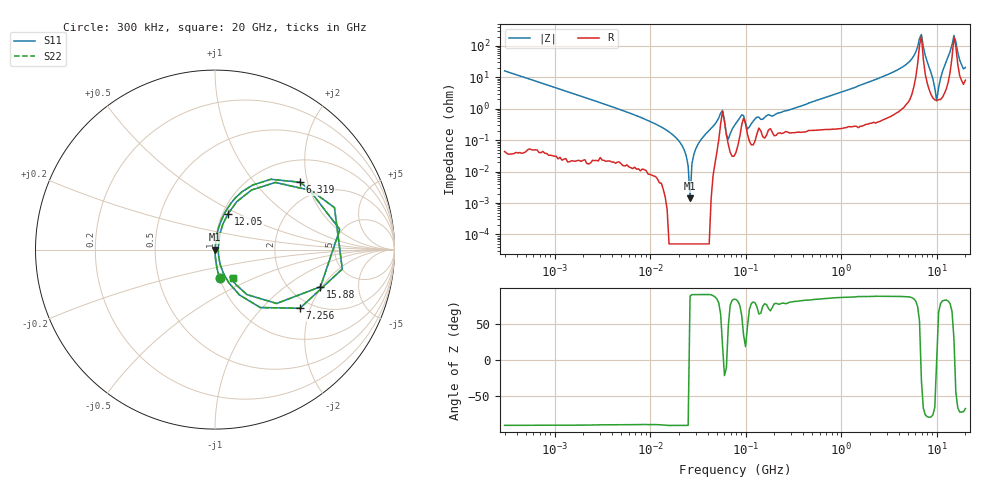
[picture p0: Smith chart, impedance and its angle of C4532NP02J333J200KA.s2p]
! S-parameter Generated by TDK Corporation
! Copyright(C) 2015 TDK Corporation.
! All Rights Reserved.
! TDK P/N: C4532NP02J333J200KA (Multilayer Ceramic Chip Capacitors)
! Property: C=33nF
! Size(LxWxT): 4.5x3.2x2mm, 0.177x0.126x0.079inches
! Model Type: s2p (Touchstone File Format Version 1.0)
! Frequency: DC=Yes Start=0.3MHz Stop=20000MHz 243points Log-sweep
! Note:
! Model Generated on Jun. 23, 2015
! Hash(MD5):
! Port Assignments:
!  1 ---| |--- 2
! Applicable Conditions:
!  Temperature = 25 degC
!  DC Bias Voltage = 0 V
!  Small Signal Operation
! Terms and conditions regarding TDK Simulation Models
! (1)This simulation model is being provided solely for informational purposes. Please refer to the specifications of the products in terms of detailed characteristics of such products.
! (2)In no event shall TDK Corporation of any of its subsidiaries be liable for any loss or damage arising, directly or indirectly,
!  From any information contained in this simulation model, including, but not limited to loss or damages arising from any inaccuracies, omissions or errors in connection with such information.
! (3)Any and all copyrights on this simulation model are owned by TDK Corporation.
!  Duplication or redistribution of this simulation model without prior written permission from TDK Corporation is prohibited.
! (4)This simulation model is subject to any modification or change without any prior notice.
! (5)Neither TDK Corporation nor any of its subsidiaries shall make any warranty, express or implied,
!  Including but not limited to the correctness, implied warranties of merchantability and fitness for a particular purpose with respect to this simulation models.
! (6)The use of this simulation model shall be deemed to have consented to the terms and conditions hereof.
# MHz S MA R 50
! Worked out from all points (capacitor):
!   242 points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, 300 kHz to 20 GHz, reference 50 ohm
!   read as one part in series: C = 32.9 nF near 314.2 kHz
!   lowest |Z| = 1.41 mohm at 26.22 MHz (marker M1)
!   series resonance near 26.12 MHz, so ESL is about 1.1 nH
!   S11 on the Smith chart (normalised r, x): 300 kHz: 1.00, -0.32; 6.319 GHz: 1.52, +1.79; 7.256 GHz: 1.74, -1.70; 12.05 GHz: 1.06, +0.44; 15.88 GHz: 2.87, -1.95; 20 GHz: 1.16, -0.38
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0.3  0.1588 -80.7  0.9869 9.1  0.9869 9.1  0.1588 -80.7
1.985118  0.02401 -88.1  0.9995 1.4  0.9995 1.4  0.02401 -88.1
12.54397  0.002832 -89.0  1 0.2  1 0.2  0.002832 -89.0
20.82636  0.000807 -91.7  1 0.0  1 0.0  0.000807 -91.7
26.22373  3.861e-05 158.5  1 -0.0  1 -0.0  3.861e-05 158.5
31.53257  0.0007173 92.8  1 -0.0  1 -0.0  0.0007173 92.8
57.40771  0.008748 18.2  0.9917 -0.2  0.9917 -0.2  0.008748 18.2
65.92025  0.001072 47.1  0.9993 -0.0  0.9993 -0.0  0.001072 47.1
79.26541  0.003439 83.0  0.9996 -0.2  0.9996 -0.2  0.003439 83.0
95.31223  0.006082 33.9  0.995 -0.2  0.995 -0.2  0.006082 33.9
104.5156  0.002269 45.9  0.9984 -0.1  0.9984 -0.1  0.002269 45.9
500.8786  0.0167 82.0  0.9978 -0.9  0.9978 -0.9  0.0167 82.0
3165.055  0.1264 80.3  0.9866 -7.3  0.9866 -7.3  0.1264 80.3
6318.653  0.6038 38.5  0.6456 -35.4  0.6456 -35.4  0.6038 38.5
6928.783  0.7174 -8.7  0.3086 19.5  0.3086 19.5  0.7174 -8.7
7255.597  0.5751 -34.6  0.616 31.6  0.616 31.6  0.5751 -34.6
9135.962  0.08672 -70.7  0.9748 4.8  0.9748 4.8  0.08672 -70.7
10018.13  0.01783 -2.4  0.9822 -0.0  0.9822 -0.0  0.01783 -2.4
12046.24  0.2125 70.0  0.9484 -12.2  0.9484 -12.2  0.2125 70.0
14484.93  0.6225 32.1  0.5745 -34.6  0.5745 -34.6  0.6225 32.1
15883.6  0.6231 -19.4  0.4549 25.1  0.4549 25.1  0.6231 -19.4
20000  0.1874 -56.9  0.9112 9.9  0.9112 9.9  0.1874 -56.9
